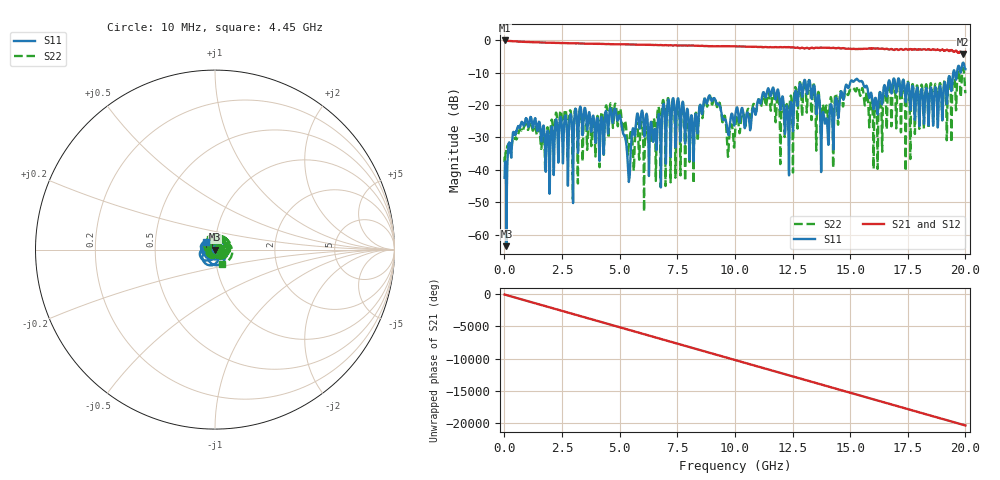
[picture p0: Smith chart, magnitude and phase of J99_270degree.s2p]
!Keysight Technologies,N5222A,MY51421036,A.10.65.16
!Date: Friday, March 31, 2023 15:03:25
!Correction: S11(Full 2 Port(1,2))
!S21(Full 2 Port(1,2))
!S12(Full 2 Port(1,2))
!S22(Full 2 Port(1,2))
!S2P File: Measurements: S11, S21, S12, S22:
# Hz S  dB  R 50
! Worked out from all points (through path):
!   2000 points, 10 MHz to 20 GHz, reference 50 ohm
!   highest |S21| = -0.10 dB at 10 MHz (marker M1); lowest = -4.3 dB at 19.9 GHz (marker M2)
!   group delay of S21, straight-line fit = 2.84 ns
!   lowest |S11| = -63.5 dB at 90 MHz (marker M3), VSWR 1.00, Z = 49.9 + j0.0296 ohm
!   |S11| at or under -10 dB: start of sweep to 19.47 GHz; 19.54 GHz to 19.64 GHz (100.6 MHz wide, 0.514 % of centre); 19.78784 GHz to 19.79281 GHz (4.967 MHz wide, 0.0251 % of centre)
!   |S22| runs from -52.9 to -8.6 dB; largest |S21 - S12| = 0.024
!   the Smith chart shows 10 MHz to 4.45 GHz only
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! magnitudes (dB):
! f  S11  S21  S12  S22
! 10 MHz  -42.5  -0.1  -0.1  -35.9
! 90 MHz  -63.5  -0.2  -0.2  -33.4
! 690 MHz  -26.3  -0.5  -0.5  -27.5
! 1.88 GHz  -28.1  -0.8  -0.8  -27.0
! 3.35 GHz  -23.4  -1.0  -1.0  -24.9
! 4.87 GHz  -23.7  -1.3  -1.3  -22.1
! 5.39 GHz  -42.3  -1.3  -1.3  -33.1
! 5.82 GHz  -24.2  -1.4  -1.4  -32.6
! 6.68 GHz  -23.5  -1.6  -1.5  -20.5
! 8.12 GHz  -23.1  -1.7  -1.7  -24.2
! 8.96 GHz  -18.2  -1.9  -1.8  -18.2
! 10.01 GHz  -23.9  -1.9  -1.9  -28.5
! 11.62 GHz  -15.1  -2.2  -2.2  -17.5
! 12.27 GHz  -20.4  -2.2  -2.2  -20.3
! 13.34 GHz  -18.0  -2.3  -2.3  -22.4
! 13.99 GHz  -24.7  -2.4  -2.3  -20.4
! 15.09 GHz  -12.6  -2.7  -2.7  -15.4
! 16.1 GHz  -17.8  -2.6  -2.5  -18.0
! 16.67 GHz  -12.8  -2.9  -2.8  -13.2
! 18.71 GHz  -14.6  -3.0  -2.9  -13.6
! 19.9 GHz  -7.0  -4.3  -4.0  -8.6
! 20 GHz  -9.0  -3.6  -3.5  -16.4
